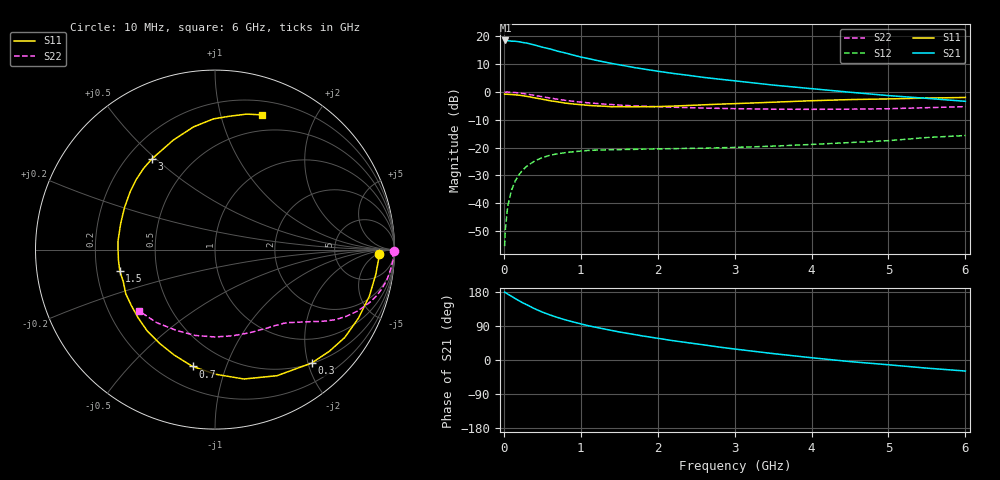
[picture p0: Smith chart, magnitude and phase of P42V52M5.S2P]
! SIEMENS Small Signal Semiconductors
! BFP182
! Si NPN RF Bipolar Junction Transistor in SOT143
! VCE = 2.5 V  IC = 2.5 mA
! Common Emitter S-Parameters:  March  1996
# GHz  S  MA  R  50
!  f  S11  S21  S12  S22
! GHz  MAG  ANG  MAG  ANG  MAG  ANG  MAG  ANG
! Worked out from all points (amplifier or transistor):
!   36 points, 10 MHz to 6 GHz, reference 50 ohm
!   highest |S21| = 18.5 dB at 20 MHz (marker M1)
!   |S21| within 3 dB of that: start of sweep to 593.1 MHz
!   unconditionally stable (mu >= 1): 2.034 GHz to 5.799 GHz
!   at 250 MHz: K = 0.14, MSG = 22.8 dB, |S12| = -27.9 dB
!   at 1.4 GHz: K = 0.73, MSG = 15.5 dB, |S12| = -20.7 dB
!   at 6 GHz: K = 0.97, MSG = 6.1 dB, |S12| = -15.7 dB
!   S11 on the Smith chart (normalised r, x): 10 MHz: 20, -6; 300 MHz: 0.51, -2.06; 700 MHz: 0.33, -0.77; 1.5 GHz: 0.30, -0.10; 3 GHz: 0.30, +0.49; 6 GHz: 0.33, +1.35
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0.01  0.9129 -1.7  8.258 179.1  0.0017 86.0  0.9951 -0.6
0.02  0.9126 -3.7  8.389 178.1  0.0034 88.5  0.9909 -1.3
0.05  0.9063 -8.8  8.314 174.0  0.0089 85.7  0.9937 -3.4
0.15  0.8858 -25.5  8.11 161.9  0.0255 75.7  0.9726 -10.0
0.2  0.8732 -34.1  7.939 156.1  0.0331 70.8  0.9558 -13.1
0.3  0.8302 -49.6  7.522 145.6  0.0465 62.6  0.9124 -18.7
0.4  0.783 -63.8  6.944 135.3  0.0575 55.3  0.8653 -23.3
0.5  0.7387 -77.4  6.358 126.5  0.0661 49.0  0.8197 -27.0
0.6  0.6946 -89.7  5.909 118.9  0.0729 43.6  0.7775 -30.1
0.7  0.6629 -100.9  5.381 112.1  0.0776 39.4  0.7377 -32.6
0.8  0.6296 -111.3  4.996 105.9  0.0811 35.7  0.7053 -34.6
0.9  0.6069 -120.5  4.59 100.5  0.0843 32.5  0.6778 -36.2
1.1  0.5728 -138.3  3.966 90.3  0.089 27.9  0.6363 -39.3
1.3  0.5547 -153.7  3.459 82.0  0.091 24.1  0.6051 -42.0
1.5  0.5437 -167.4  3.068 74.0  0.092 22.1  0.5798 -44.5
1.8  0.5424 174.8  2.598 63.6  0.0938 19.8  0.5554 -48.3
2.2  0.5558 155.2  2.147 51.0  0.0958 18.4  0.531 -54.2
3  0.6157 124.8  1.582 29.0  0.1008 18.5  0.5002 -68.3
3.5  0.653 110.8  1.327 16.9  0.1062 18.8  0.4901 -78.6
4.5  0.7282 90.7  0.987 -4.2  0.1232 19.3  0.4907 -102.8
5.5  0.775 76.9  0.766 -21.5  0.1517 17.9  0.5209 -128.6
6  0.7946 70.9  0.678 -29.1  0.1649 14.5  0.544 -141.2
